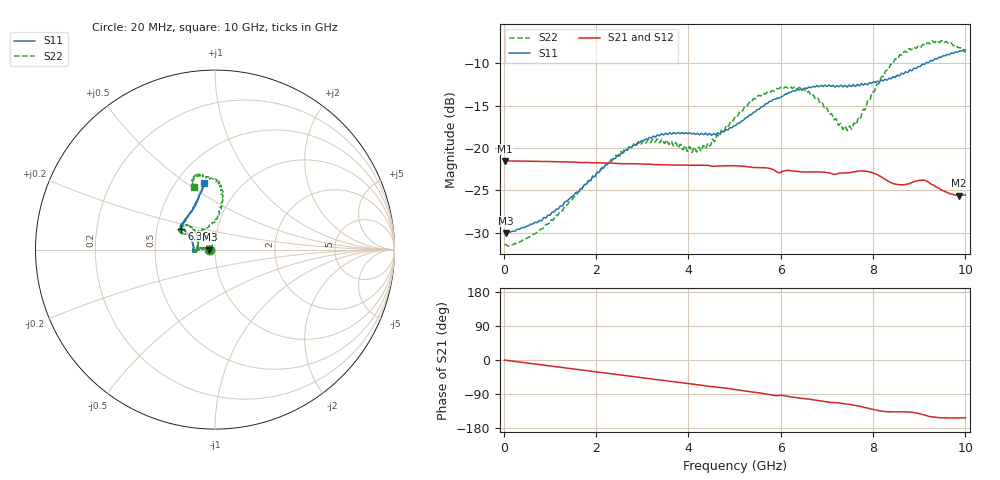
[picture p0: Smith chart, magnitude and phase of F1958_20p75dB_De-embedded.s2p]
! Integrated Device Technology
! Corporate Headquarters
! 6024 Silver Creek Valley Road
! San Jose, CA 95138  USA
! Phone:  1-408-284-8200
! Toll Free:  1-800-223-1366
! Webpage:  http://www.idt.com/
! Timing and RF Division
! 515 Groton Road, Suite 102
! Westford, MA 01886-6024
! Device:  F1958
! Description: 7-bit 0.25 dB Digital Step Attenuator
! Frequency:  0.001 -  6.000 GHz
! Package:  4x4 mm Thin QFN Plastic Package: 24 pin
! Ports:  2 RF, 12 DC
!  Pin  1  = D0
!  Pin  2  = VDD
!  Pin  3  = VMODE
!  Pin  4  = GND
!  Pin  5  = RF1  =  Port 1
!  Pin  6  = GND
!  Pin  7  = GND
!  Pin  8  = GND
!  Pin  9  = GND
!  Pin 10  = GND
!  Pin 11  = GND
!  Pin 12  = GND
!  Pin 13  = GND
!  Pin 14  = RF2  =  Port 2
!  Pin 15  = GND
!  Pin 16  = LE
!  Pin 17  = CLK
!  Pin 18  = DATA
!  Pin 19  = D6
!  Pin 20  = D5
!  Pin 21  = D4
!  Pin 22  = D3
!  Pin 23  = D2
!  Pin 24  = D1
! State:  83
! Atten State:  20.75 dB
! Voltage:  +3.30 Volts
! Current:  0.258 mA
! Data:  The device was measured on a F1958 evaluation board which has
!  individual transmission lines to the RF pins.  Data was collected
!  using a calibrated network analyzer.  The evaluation board was
!  de-embedded using Automatic Fixture Removal (AFR).
!  The reference plane is the edge of the package pin.
! Misc:
!  Action Tracker AT0419
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# GHz S dB R 50
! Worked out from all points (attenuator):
!   500 points, 20 MHz to 10 GHz, reference 50 ohm
!   highest |S21| = -21.52 dB at 20 MHz (marker M1); lowest = -25.6 dB at 9.86 GHz (marker M2)
!   lowest |S11| = -30.0 dB at 40 MHz (marker M3), VSWR 1.06, Z = 46.9 - j0.04 ohm
!   |S11| at or under -10 dB: start of sweep to 9.142 GHz
!   |S22| runs from -31.6 to -7.3 dB; largest |S21 - S12| = 0.00033
!   S11 on the Smith chart (normalised r, x): 20 MHz: 0.94, -0.00; 6.36 GHz: 0.67, +0.16; 10 GHz: 0.68, +0.59
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0.02  -30.01 -178.9  -21.52 -0.4  -21.52 -0.4  -31.43 -178.6
0.04  -30.04 -179.2  -21.52 -0.7  -21.52 -0.7  -31.39 -177.9
0.84  -28.44 171.2  -21.60 -13.3  -21.59 -13.3  -29.53 178.2
1.7  -24.77 171.2  -21.72 -26.6  -21.71 -26.5  -24.77 176.4
2.6  -20.52 177.0  -21.86 -40.5  -21.83 -40.5  -20.29 -179.1
3.36  -18.55 -175.7  -21.98 -52.4  -21.98 -52.5  -19.25 -171.8
4.24  -18.45 -179.2  -22.03 -65.7  -22.04 -65.8  -19.95 165.9
4.64  -18.21 171.7  -22.14 -71.7  -22.15 -71.7  -18.48 148.0
5.02  -17.37 160.7  -22.09 -78.0  -22.11 -78.1  -16.20 137.6
5.58  -15.14 150.5  -22.34 -87.6  -22.35 -87.6  -13.79 138.0
6.36  -13.13 147.9  -22.77 -99.7  -22.79 -99.7  -13.08 151.2
6.68  -12.80 146.4  -22.83 -104.4  -22.84 -104.3  -13.77 152.2
7.3  -12.60 140.7  -22.97 -114.1  -22.97 -114.0  -17.13 130.9
7.5  -12.63 138.0  -22.91 -117.3  -22.91 -117.2  -17.44 112.5
7.68  -12.59 135.1  -22.73 -121.1  -22.72 -121.1  -16.42 95.7
7.9  -12.41 128.8  -22.80 -127.5  -22.79 -127.6  -14.39 86.8
8.34  -11.80 119.0  -23.96 -136.8  -23.96 -136.9  -10.67 81.6
8.68  -11.17 112.2  -24.36 -137.0  -24.33 -136.7  -8.59 86.2
9.06  -10.15 106.7  -23.82 -143.5  -23.84 -143.6  -7.92 94.3
9.26  -9.67 104.6  -24.28 -149.7  -24.27 -149.7  -7.50 99.2
9.86  -8.60 99.7  -25.62 -152.7  -25.64 -152.6  -8.19 108.2
10  -8.47 99.7  -25.55 -153.0  -25.55 -152.9  -8.71 109.0
